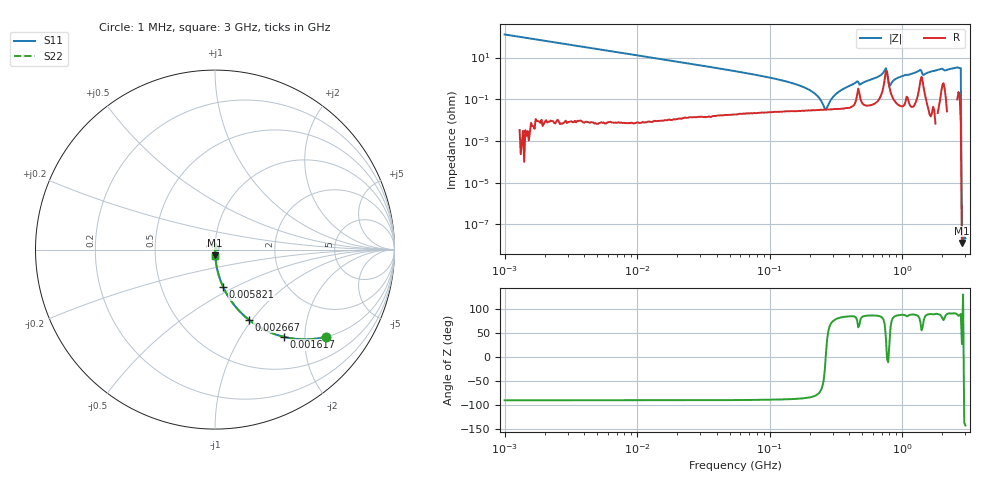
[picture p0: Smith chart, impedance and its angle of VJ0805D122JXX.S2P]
! VJ0805D122JXX
! DATE
! CORRECTED  DATA
# Hz  S  MA  R  50
!Freq	S11M	S11A	S21M	S21A	S12M	S12A	S22M	S22A
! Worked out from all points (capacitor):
!   401 points, 1 MHz to 3 GHz, reference 50 ohm
!   read as one part in series: C = 1.25 nF near 1.041 MHz
!   lowest |Z| = 12.8 nohm at 2.825 GHz (marker M1)
!   series resonance near 265 MHz, so ESL is about 290 pH
!   S11 on the Smith chart (normalised r, x): 1 MHz: 1.00, -2.55; 1.617 MHz: 1.00, -1.58; 2.667 MHz: 1.00, -0.96; 5.821 MHz: 1.00, -0.44; 3 GHz: 1.00, -0.07
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1000000  0.7875 -38.1  0.6165 52.0  0.6165 52.0  0.7875 -38.1
1616692  0.6199 -51.7  0.7846 38.3  0.7846 38.3  0.6199 -51.7
2666535  0.432 -64.4  0.9018 25.6  0.9018 25.6  0.432 -64.4
3823119  0.3168 -71.5  0.9484 18.5  0.9484 18.5  0.3168 -71.5
5820586  0.2142 -77.6  0.9767 12.4  0.9767 12.4  0.2142 -77.6
1.461624e7  0.08673 -85.0  0.9961 5.0  0.9961 5.0  0.08673 -85.0
5.587962e7  0.02176 -88.3  0.9996 1.2  0.9996 1.2  0.02176 -88.3
1.348146e8  0.00701 -87.4  0.9997 0.4  0.9997 0.4  0.00701 -87.4
2.094008e8  0.002312 -82.7  0.9997 0.1  0.9997 0.1  0.002312 -82.7
2.662515e8  0.000318 8.8  0.9997 -0.0  0.9997 -0.0  0.000318 8.8
3.188066e8  0.00185 79.5  0.9997 -0.1  0.9997 -0.1  0.00185 79.5
4.480278e8  0.00644 82.1  0.9991 -0.4  0.9991 -0.4  0.00644 82.1
4.951867e8  0.005742 82.6  0.9993 -0.3  0.9993 -0.3  0.005742 82.6
7.38967e8  0.0244 66.1  0.9904 -1.3  0.9904 -1.3  0.0244 66.1
8.005644e8  0.004263 26.3  0.9962 -0.1  0.9962 -0.1  0.004263 26.3
8.332625e8  0.006147 75.2  0.9984 -0.3  0.9984 -0.3  0.006147 75.2
9.395906e8  0.01104 86.6  0.9994 -0.6  0.9994 -0.6  0.01104 86.6
1.320433e9  0.02195 84.0  0.998 -1.3  0.998 -1.3  0.02195 84.0
1.488926e9  0.01624 83.7  0.9983 -0.9  0.9983 -0.9  0.01624 83.7
1.931433e9  0.0275 86.5  0.9987 -1.6  0.9987 -1.6  0.0275 86.5
2.825159e9  0.03178 -89.9  1.001 -1.8  1.001 -1.8  0.03178 -89.9
3e9  0.03445 -88.5  1.001 -2.0  1.001 -2.0  0.03445 -88.5
